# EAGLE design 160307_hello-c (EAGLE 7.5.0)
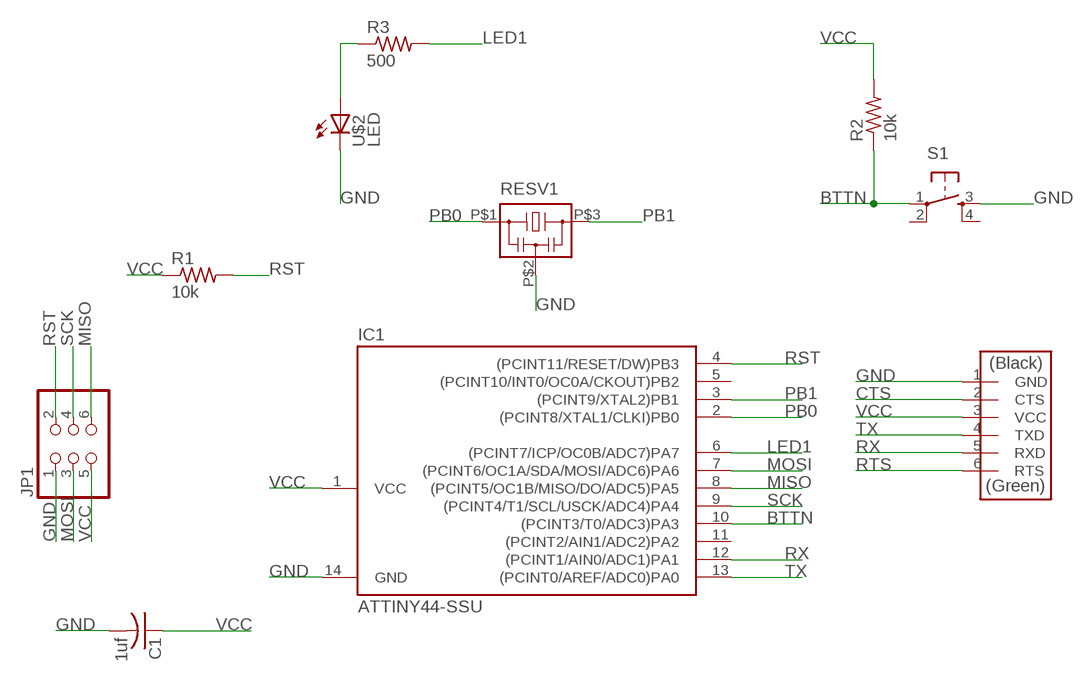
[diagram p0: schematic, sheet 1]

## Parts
C1  1uf  C-USC1206  [C1206]
IC1  ATTINY44-SSU  [SOIC14]
JP1  PINHD-2X3-SMD  [2X03SMD]
R1  10k  RES-US1206  [R1206]
R2  10k  RES-US1206  [R1206]
R3  500  RES-US1206  [R1206]
RESV1  RESONATOR-VOLT  [VOLT]
S1  6MM_SWITCH6MM_SWITCH  [6MM_SWITCH]
U$1  FTDI-SMD-HEADER  [1X06SMD]
U$2  LED  [LED1206]

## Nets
BTTN: IC1.10((PCINT3/T0/ADC3)PA3) R2.1 S1.1(P)
CTS: U$1.2(CTS)
GND: C1.2 IC1.14(GND) JP1.1 RESV1.P$2 S1.3(S) U$1.1(GND) U$2.2(C)
LED1: IC1.6((PCINT7/ICP/OC0B/ADC7)PA7) R3.2
MISO: IC1.8((PCINT5/OC1B/MISO/DO/ADC5)PA5) JP1.6
MOSI: IC1.7((PCINT6/OC1A/SDA/MOSI/ADC6)PA6) JP1.3
N$1: R3.1 U$2.1(A)
PB0: IC1.2((PCINT8/XTAL1/CLKI)PB0) RESV1.P$1
PB1: IC1.3((PCINT9/XTAL2)PB1) RESV1.P$3
RST: IC1.4((PCINT11/RESET/DW)PB3) JP1.2 R1.2
RTS: U$1.6(RTS)
RX: IC1.12((PCINT1/AIN0/ADC1)PA1) U$1.5(RXD)
SCK: IC1.9((PCINT4/T1/SCL/USCK/ADC4)PA4) JP1.4
TX: IC1.13((PCINT0/AREF/ADC0)PA0) U$1.4(TXD)
VCC: C1.1 IC1.1(VCC) JP1.5 R1.1 R2.2 U$1.3(VCC)
Unconnected: IC1.5((PCINT10/INT0/OC0A/CKOUT)PB2) IC1.11((PCINT2/AIN1/ADC2)PA2) S1.2(P1) S1.4(S1)

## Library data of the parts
C1 = rcl:C-US: CAPACITOR, American symbol
IC1 = fab:ATTINY44
JP1 = fab:PINHD-2X3-SMD: PIN HEADER
R1-R3 = fab:RES-US: Resistor (US Symbol)
RESV1 = Volt:RESONATOR-VOLT
S1 = fab:6MM_SWITCH: OMRON SWITCH
U$1 = fab:FTDI-SMD-HEADER
U$2 = fab:LED: LED

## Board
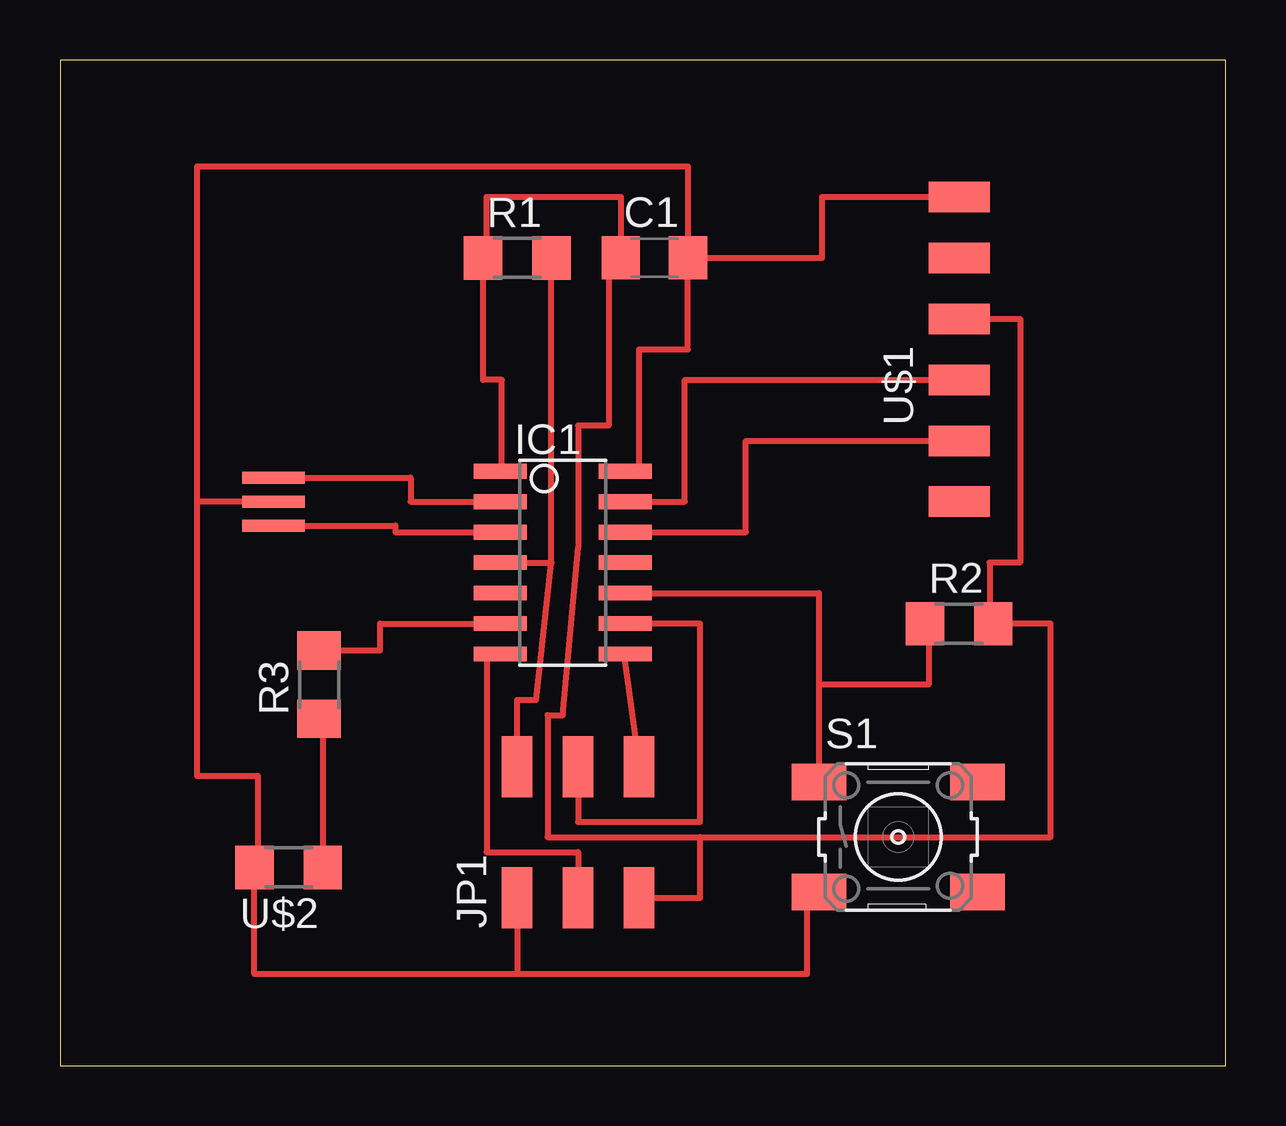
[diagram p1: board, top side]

Size 48.57 x 41.9 mm. Coordinates in mm from the lower left corner, seen from the top.
Outline: 0,0 48.57,0 48.57,41.9 0,41.9 0,0
Copper layers (1*16): Top 0.035mm / dielectric 1.5mm / Bottom 0.035mm
Design rules "default": minimum track width 10mil, minimum drill 24mil, track to track 8mil, track to pad 8mil, pad to pad 8mil, via to via 8mil, smd to smd 8mil, copper to edge 40mil, drill to drill 8mil, minimum pad ring 10mil, minimum via ring 8mil, stop-mask expansion 4mil, vias tented up to drill 0mil, thermal gap 10mil

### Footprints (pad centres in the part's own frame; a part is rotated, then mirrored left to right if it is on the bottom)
C1206 = smd 1.6 x 1.8: 1 -1.4,0; 2 1.4,0
SOIC14 = smd 0.61 x 2.21: 1 -3.81,-2.603; 2 -2.54,-2.603; 3 -1.27,-2.603; 4 0,-2.603; 5 1.27,-2.603; 6 2.54,-2.603; 7 3.81,-2.603; 8 3.81,2.603; 9 2.54,2.603; 10 1.27,2.603; 11 0,2.603; 12 -1.27,2.603; 13 -2.54,2.603; 14 -3.81,2.603
2X03SMD = smd 2.54 x 1.27: 1 -2.54,2.54; 2 2.92,2.54; 3 -2.54,0; 4 2.92,0; 5 -2.54,-2.54; 6 2.92,-2.54
R1206 = smd 1.6 x 1.803: 1 -1.422,0; 2 1.422,0
VOLT = smd 0.5 x 2.6: P$1 -1,0; P$2 0,0; P$3 1,0
6MM_SWITCH = smd 2.286 x 1.524: 1 -3.302,2.286; 2 3.302,2.286; 3 -3.302,-2.286; 4 3.302,-2.286
1X06SMD = smd 2.54 x 1.27: 1 0,6.35; 2 0,3.81; 3 0,1.27; 4 0,-1.27; 5 0,-3.81; 6 0,-6.35
LED1206 = smd 1.6 x 1.803: 1 -1.422,0; 2 1.422,0

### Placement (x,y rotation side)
C1  24.77,33.66 0 top
IC1  20.96,20.95 270 top
JP1  21.59,9.53 90 top
R1  19.05,33.66 0 top
R2  37.47,18.41 0 top
R3  10.79,15.88 90 top
RESV1  8.89,23.49 270 top
S1  34.93,9.53 0 top
U$1  37.47,29.84 0 top
U$2  9.53,8.26 180 top

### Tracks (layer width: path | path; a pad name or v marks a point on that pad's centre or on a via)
BTTN
  Top 0.254: R2.1 36.2,18.41 36.2,15.88 31.62,15.88 | 31.62,15.88 S1.1 | IC1.10 31.62,19.69 31.62,15.88
GND
  Top 0.254: C1.2 31.75,33.66 31.75,36.2 U$1.1 | IC1.14 24.13,24.77 24.13,29.84 26.17,29.84 C1.2 | S1.3 31.11,7.24 31.11,3.81 19.05,3.81 | JP1.1 19.05,3.81 | 19.05,3.81 8.1,3.81 U$2.2 8.25,8.26 8.25,12.07 5.71,12.07 5.71,23.49 | RESV1.P$2 5.71,23.49 | 5.71,23.49 5.71,37.47 26.17,37.47 C1.2
LED1
  Top 0.254: R3.2 13.34,17.3 13.34,18.41 IC1.6
MISO
  Top 0.254: IC1.8 23.5,17.15 JP1.6
MOSI
  Top 0.254: IC1.7 17.78,17.15 17.78,8.89 21.59,8.89 JP1.3
N$1
  Top 0.254: R3.1 10.95,14.45 U$2.1
PB0
  Top 0.254: RESV1.P$1 14.61,24.49 14.61,23.49 IC1.2
PB1
  Top 0.254: RESV1.P$3 13.97,22.49 13.97,22.23 IC1.3
RST
  Top 0.254: JP1.2 19.05,15.24 19.84,15.24 20.47,20.95 | 20.47,20.95 R1.2 | IC1.4 20.47,20.95
RX
  Top 0.254: IC1.12 28.57,22.23 28.57,26.04 U$1.5
SCK
  Top 0.254: JP1.4 21.59,10.16 26.67,10.16 26.67,18.41 IC1.9
TX
  Top 0.254: IC1.13 26.04,23.49 26.04,28.58 U$1.4
VCC
  Top 0.254: U$1.3 40.01,31.12 40.01,20.95 38.73,20.95 38.73,18.41 R2.2 41.28,18.41 41.28,9.53 26.67,9.53 | JP1.5 26.67,6.98 26.67,9.53 | IC1.1 18.42,24.77 18.42,28.58 17.63,28.58 R1.1 17.78,33.66 17.78,36.2 23.36,36.2 C1.1 22.86,33.66 22.86,26.67 21.59,26.67 21.59,21.59 20.96,14.61 20.32,14.61 20.32,9.53 26.67,9.53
